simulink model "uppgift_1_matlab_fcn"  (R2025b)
settings: Solver=VariableStepAuto  StartTime=0.0  StopTime=10.0  RelTol=1e-3

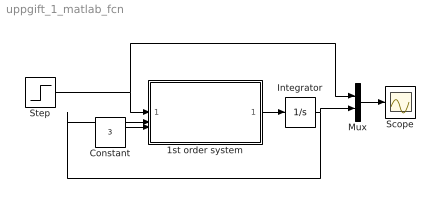
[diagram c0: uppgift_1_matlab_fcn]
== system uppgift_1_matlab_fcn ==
  1st order system : MATLAB Function  TreatAsAtomicUnit=on
  Constant : Constant  Value=3
  Integrator : Integrator
  Mux : Mux  Inputs=2
  Scope : Scope
  Step : Step  SampleTime=0
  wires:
  Mux/1 -> Scope/1
  Integrator/1 -> 1st order system/2(actual), Mux/2
  Step/1 -> Mux/1, 1st order system/1(ref)
  1st order system/1(alpha) -> Integrator/1
  Constant/1 -> 1st order system/3(tau)

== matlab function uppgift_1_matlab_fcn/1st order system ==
function alpha = fcn(ref, actual, tau)
error = ref - actual;

alpha =  error/tau;
